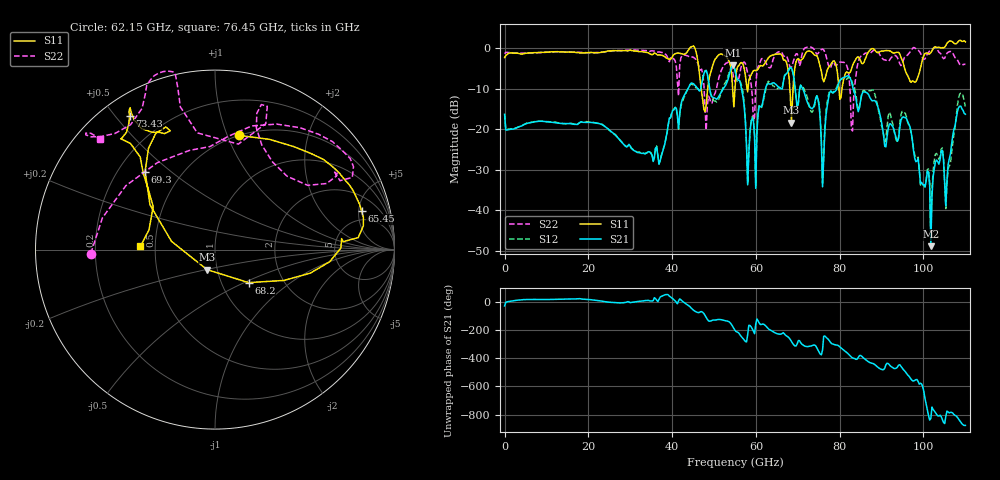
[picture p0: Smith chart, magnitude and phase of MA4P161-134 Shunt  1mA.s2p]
!Keysight Technologies,N5247B,US61255204,A.15.70.20
!Date: Friday, October 21, 2022 14:11:01
!Correction: S11(C  4-Port  )
!S31(C  4-Port  )
!S13(C  4-Port  )
!S33(C  4-Port  )
!S2P File: Measurements: S11, S31, S13, S33:
# Hz S  dB  R 50
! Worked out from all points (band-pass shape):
!   401 points, 10 MHz to 110 GHz, reference 50 ohm
!   highest |S21| = -4.30 dB at 54.46 GHz (marker M1); lowest = -48.8 dB at 101.8 GHz (marker M2)
!   |S21| within 3 dB of the highest: 53.46 GHz to 55.44 GHz (1.983 GHz wide, 3.64 % of centre); 66.74 GHz to 69.04 GHz (2.3 GHz wide, 3.39 % of centre)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
!   lowest |S11| = -18.4 dB at 68.48 GHz (marker M3), VSWR 1.27, Z = 44.7 - j10.1 ohm
!   |S11| at or under -10 dB: 46.93 GHz to 48.5 GHz (1.57 GHz wide, 3.29 % of centre); 54.45 GHz to 55 GHz (554.8 MHz wide, 1.01 % of centre); 68.09 GHz to 68.87 GHz (777.8 MHz wide, 1.14 % of centre)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
!   |S22| runs from -20.5 to 0.3 dB; largest |S21 - S12| = 0.16
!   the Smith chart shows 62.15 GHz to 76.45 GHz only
!   S11 on the Smith chart (normalised r, x): 62.15 GHz: 0.50, +1.10; 65.45 GHz: 3.57, +5.38; 68.2 GHz: 1.34, -0.53; 69.3 GHz: 0.31, +0.41; 73.43 GHz: 0.08, +0.54; 76.45 GHz: 0.41, +0.02
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1e7  -2.36 -174.9  -16.34 -28.3  -16.29 -28.1  -1.41 -174.9
1.843332e10  -1.20 130.7  -18.20 20.6  -18.21 20.5  -1.06 140.5
3.685665e10  -1.69 126.3  -28.64 18.6  -28.51 18.9  -0.95 133.7
4.565585e10  -0.71 52.5  -9.42 -69.1  -9.79 -67.5  -2.81 27.2
5.445505e10  -10.09 98.3  -4.30 -174.0  -4.37 -173.7  -5.96 127.5
5.5005e10  -9.98 -177.6  -5.34 158.8  -5.56 158.4  -8.31 147.9
5.802972e10  -10.83 159.3  -33.72 127.8  -33.42 127.1  -6.15 167.6
6.077948e10  -4.70 149.6  -14.32 -149.2  -13.97 -150.2  -4.15 -121.9
6.215435e10  -3.74 78.0  -10.51 -164.8  -11.22 -159.3  -3.19 -178.2
6.545405e10  -1.47 14.8  -9.67 132.0  -9.70 154.0  -0.93 37.9
6.82038e10  -11.62 -44.5  -4.72 93.0  -4.88 90.2  -4.84 45.5
6.847878e10  -18.41 -111.5  -4.89 79.7  -5.09 77.4  -4.67 56.7
6.93037e10  -4.68 131.9  -9.41 47.7  -9.15 47.1  -2.00 72.9
7.342832e10  -1.07 122.6  -14.94 50.7  -15.78 49.0  0.08 111.0
7.645305e10  -7.62 177.5  -20.33 118.4  -19.33 130.6  -1.00 136.0
8.085265e10  -8.15 -76.0  -7.26 20.5  -7.68 20.9  -3.51 -143.8
8.305245e10  -4.35 -45.6  -9.30 -37.1  -8.76 -20.8  -20.45 9.9
8.607718e10  -2.78 6.3  -10.87 -47.4  -10.72 -46.1  -1.28 -14.8
9.185165e10  -0.67 71.6  -18.73 -85.9  -15.78 -82.7  -3.02 67.1
9.762612e10  -8.20 177.9  -25.30 158.4  -24.87 156.7  0.13 166.0
1.017508e11  -1.16 -88.1  -48.84 -107.9  -46.52 -103.7  -0.49 -124.6
1.1e11  1.54 8.3  -16.31 -156.7  -14.42 -161.3  -4.05 16.7
